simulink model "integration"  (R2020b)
settings: Solver=FixedStepAuto  StartTime=0.0  StopTime=10  FixedStep=0.02  RelTol=1e-3
libraries: sldrtlib x1

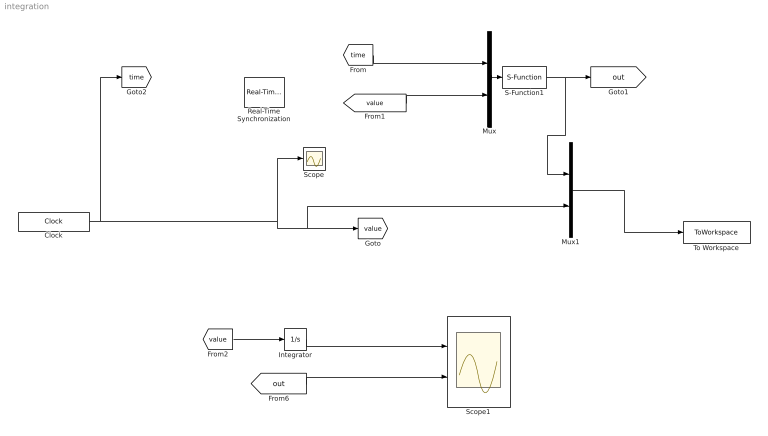
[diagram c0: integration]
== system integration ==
  Clock : Clock
  Integrator : Integrator
  Mux : Mux  Inputs=2
  Mux1 : Mux  Inputs=2
  Real-Time Synchronization : sldrtlib/Real-Time Synchronization  SampleTime=0.02  MaxMissedTicks=inf  ShowMissedTicks=off  YieldWhenWaiting=off
  S-Function1 : S-Function  FunctionName=modbusComintegral  SFunctionDeploymentMode=off  EnableBusSupport=off
  Scope : Scope
  Scope1 : Scope  NumInputPorts=2
  To Workspace : ToWorkspace  VariableName=simout  SampleTime=-1
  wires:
  S-Function1/1 -> Mux1/1, [out]
  [out] -> Scope1/2
  [value] -> Mux/2
  Mux/1 -> S-Function1/1
  [time] -> Mux/1
  [value] -> Integrator/1
  Integrator/1 -> Scope1/1
  Mux1/1 -> To Workspace/1
  Clock/1 -> Mux1/2, [value], Scope/1, [time]
